//{{V2}}
FUNCTION_BLOCK FB33
TITLE=Set Homing Parameter
//*****************************************************************************
//* maxon motor ag
//* R&D
//* all rights reserved
//*****************************************************************************
//* Summary:  Set all homing parameters
//*
//* Remarks:
//*
//* Created under: STEP7 REV5.2+SP1
//*****************************************************************************
//* History:
//* 18.05.2004 | INA   first release
//*
//*
//*****************************************************************************
//


AUTHOR:INA
FAMILY:HomingMo
NAME:SetHoPa
VERSION:00.01


VAR_INPUT
       Write:BOOL //A rising edge start the command
       NodeID:BYTE //Adress of the maxon device
       HomingAcceleration:DWORD //Acceleration for Homing Profile
       SpeedSwitch:DWORD //Speed during search for switch
       SpeedIndex:DWORD //Speed during search for index signal
       HomeOffset:DINT //Home Offset after Homing
       CurrentThreshold:WORD //Current Threshold for Homing Method -3 and -4
       HomePosition:DINT //Home position value
END_VAR

VAR_OUTPUT
       Done:BOOL //Data valid flag is TRUE if data were available
       Err:BOOL //Error flag is TRUE if an Error has occured, see ErrNo for more details
       ErrNo:DINT //Contains detailed error information
END_VAR

VAR_IN_OUT
END_VAR

VAR
       xEdgeMerker:BOOL //Edge Merker
       xEdgeFlag:BOOL //Edge Flag
       xStep:INT
END_VAR

VAR_TEMP
END_VAR
BEGIN

NETWORK
TITLE= Activate the service function
//{{a}}
//

// SDO Write "Set Homing Parameter"

       U    #Write
       FP   #xEdgeFlag                   // recognize a positiv edge of the Read signal
       =    #xEdgeMerker                 // and set the xEdgeMerker for one cycle to true

       L    #xStep
       L    0
       ==I
       U    #xEdgeMerker
       SPB  nstp                         // iStep = 1 -> fnc1

       L    #xStep                       // jump list
       SPL  List
       SPA  rdef
       SPA  fnc1
       SPA  fncE
List  :SPA  rdef

rdef  :NOP  0
       R    #Done                        // reset Done
       R    #Err
       L    0
       T    #xStep                       // iStep = 0
       SPA  end

fnc1  :NOP  0
       CALL FC16
         NodeID:=#NodeID
         Index:=DW#16#00006099
         SubIndex:=DW#16#00000002
         ValueIn:=#SpeedIndex
         RET_VAL:=#Done
         Err:=#Err
         ErrNo:=#ErrNo

       L    1
       U    #Err
       SPB  fncE

       NOP  0
       CALL FC16
         NodeID:=#NodeID
         Index:=DW#16#0000609A
         SubIndex:=DW#16#00000000
         ValueIn:=#HomingAcceleration
         RET_VAL:=#Done
         Err:=#Err
         ErrNo:=#ErrNo

       L    1
       U    #Err
       SPB  fncE

       NOP  0
       CALL FC16
         NodeID:=#NodeID
         Index:=DW#16#00006099
         SubIndex:=DW#16#00000001
         ValueIn:=#SpeedSwitch
         RET_VAL:=#Done
         Err:=#Err
         ErrNo:=#ErrNo

       L    1
       U    #Err
       SPB  fncE

       NOP  0
       CALL FC13
         NodeID:=#NodeID
         Index:=DW#16#0000607C
         SubIndex:=DW#16#00000000
         ValueIn:=#HomeOffset
         RET_VAL:=#Done
         Err:=#Err
         ErrNo:=#ErrNo

       L    1
       U    #Err
       SPB  fncE

       NOP  0
       CALL FC15
         NodeID:=#NodeID
         Index:=DW#16#00002080
         SubIndex:=DW#16#00000000
         ValueIn:=#CurrentThreshold
         RET_VAL:=#Done
         Err:=#Err
         ErrNo:=#ErrNo

       L    1
       U    #Err
       SPB  fncE

       NOP  0
       CALL FC13
         NodeID:=#NodeID
         Index:=DW#16#00002081
         SubIndex:=DW#16#00000000
         ValueIn:=#HomePosition
         RET_VAL:=#Done
         Err:=#Err
         ErrNo:=#ErrNo

fncE  :NOP  0
       L    0
       T    #xStep
       SPA  end

nstp  :NOP  0
       L    #xStep
       INC            1
       T    #xStep

end   :NOP  0
END_FUNCTION_BLOCK
